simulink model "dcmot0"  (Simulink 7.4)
settings: Solver=ode45  StartTime=0.0  StopTime=1.6  MaxStep=0.004  RelTol=1e-3

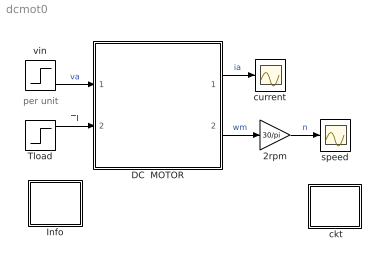
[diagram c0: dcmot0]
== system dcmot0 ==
  note: per unit
  " ckt" : Subsystem
  2rpm : Gain  Gain=30/pi  ParameterDataType=sfix(16)  ParameterScaling=2^0  OutDataType=sfix(16)  OutScaling=2^0
  DC  MOTOR : Subsystem  mask(Block diagram model of a DC motor.){La=0.03, J=0.6, Bm=0.1, K=1.85, Ra=0.60, Vr=240, Tr=30, va=1.0, Tl=1.0}
      mask prompts: La "Armature inductance [H]"; J "Moment of inertia [Kg.m^2]"; Bm "Frictional torque coefficient [N.m/rad/s]"; K "Electromechanical coupling coefficient [N.m/A]"; Ra "Armature resistance [ohm]"; Vr "Rated voltage [V]"; Tr "Rated torque [N.m]"; va "Initial voltage va [pu]"; Tl "Initial load torque Tl [pu]"
      mask help: Parameter va must be equal to the initial value of the step function vin... Parameter Tl must be equal to the initial value of the step function Tload.
      mask init:
      | %Steady-state initial operation
      | %va must be equal to the initial value of the step function vin
      | %Tl must be equal to the initial value of the step functiom Tload
      | C=[Ra K;K -Bm];
      | y0=[va*Vr;Tl*Tr];
      | x0=C\y0;
      | ia0=x0(1);
      | wm0=x0(2);
  Info : Subsystem
  Tload : Step  Time=0.2  Before=1  After=1/2  SampleTime=0
  current : Scope
  speed : Scope
  vin : Step  Time=.8  Before=1  After=[0.75 0.5]  SampleTime=0
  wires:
  vin/1 -> DC  MOTOR/1(va)  "va"
  Tload/1 -> DC  MOTOR/2(Tl)  "Tl"
  DC  MOTOR/1(ia) -> current/1  "ia"
  DC  MOTOR/2(wm) -> 2rpm/1  "wm"
  2rpm/1 -> speed/1  "n"

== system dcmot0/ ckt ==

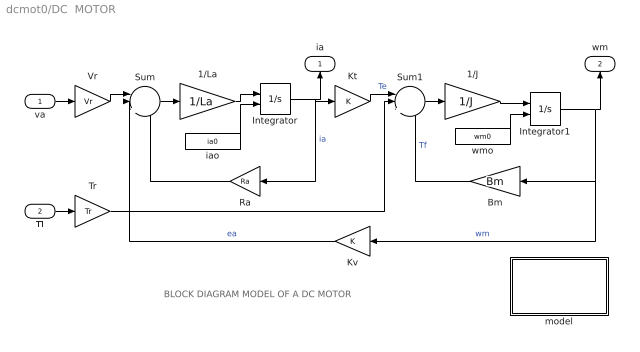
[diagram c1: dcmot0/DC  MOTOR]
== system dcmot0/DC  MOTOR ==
  note: BLOCK DIAGRAM MODEL OF A DC MOTOR
  va : Inport  OutDataType=sfix(16)  OutScaling=2^0
  Tl : Inport  Port=2  OutDataType=sfix(16)  OutScaling=2^0
  1/J : Gain  Gain=1/J  ParameterDataType=sfix(16)  ParameterScaling=2^0  OutDataType=sfix(16)  OutScaling=2^0
  1/La : Gain  Gain=1/La  ParameterDataType=sfix(16)  ParameterScaling=2^0  OutDataType=sfix(16)  OutScaling=2^0
  Bm : Gain  Gain=Bm  ParameterDataType=sfix(16)  ParameterScaling=2^0  OutDataType=sfix(16)  OutScaling=2^0
  Integrator : Integrator  InitialConditionSource=external  InitialCondition=16.2162
  Integrator1 : Integrator  InitialConditionSource=external  InitialCondition=98.5245
  Kt : Gain  Gain=K  ParameterDataType=sfix(16)  ParameterScaling=2^0  OutDataType=sfix(16)  OutScaling=2^0
  Kv : Gain  Gain=K  ParameterDataType=sfix(16)  ParameterScaling=2^0  OutDataType=sfix(16)  OutScaling=2^0
  Ra : Gain  Gain=Ra  ParameterDataType=sfix(16)  ParameterScaling=2^0  OutDataType=sfix(16)  OutScaling=2^0
  Sum : Sum  Inputs=||+--  OutDataType=sfix(16)  OutScaling=2^0
  Sum1 : Sum  Inputs=||+--  OutDataType=sfix(16)  OutScaling=2^0
  Tr : Gain  Gain=Tr  ParameterDataType=sfix(16)  ParameterScaling=2^0  OutDataType=sfix(16)  OutScaling=2^0
  Vr : Gain  Gain=Vr  ParameterDataType=sfix(16)  ParameterScaling=2^0  OutDataType=sfix(16)  OutScaling=2^0
  iao : Constant  Value=ia0  OutDataType=sfix(16)  OutScaling=2^0
  model : Subsystem
  wmo : Constant  Value=wm0  OutDataType=sfix(16)  OutScaling=2^0
  ia : Outport
  wm : Outport  Port=2
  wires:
  Kv/1 -> Sum/2  "ea"
  Ra/1 -> Sum/3
  Kt/1 -> Sum1/1  "Te"
  Bm/1 -> Sum1/3  "Tf"
  Sum/1 -> 1/La/1
  1/La/1 -> Integrator/1
  Integrator/1 -> Ra/1, Kt/1, ia/1  "ia"
  Sum1/1 -> 1/J/1
  1/J/1 -> Integrator1/1
  Integrator1/1 -> Bm/1, Kv/1, wm/1  "wm"
  va/1 -> Vr/1
  Tl/1 -> Tr/1
  iao/1 -> Integrator/2
  wmo/1 -> Integrator1/2
  Vr/1 -> Sum/1
  Tr/1 -> Sum1/2

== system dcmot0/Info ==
  note: This demo simulates the running of a DC motor with constant field or pm excitation. (5 hp 240V 1200 rpm) (rated torque Tr = 30 N.m) The motor is initially running in steady state when the load torque is suddenly changed; a little later the applied voltage is also modified.

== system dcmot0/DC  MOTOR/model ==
  note: Electrical system equation: va = Ra.ia + La.dia/dt + ea where ea = K.wm Mechanical system equation: Te = J.dwm/dt + Tl.signum(wm) + f(wm) where Te = K.ia
  note: Mathematical model of the dc machine
